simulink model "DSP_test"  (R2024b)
settings: Solver=VariableStepAuto  StartTime=0.0  StopTime=50  RelTol=1e-3
libraries: hdlsllib x1

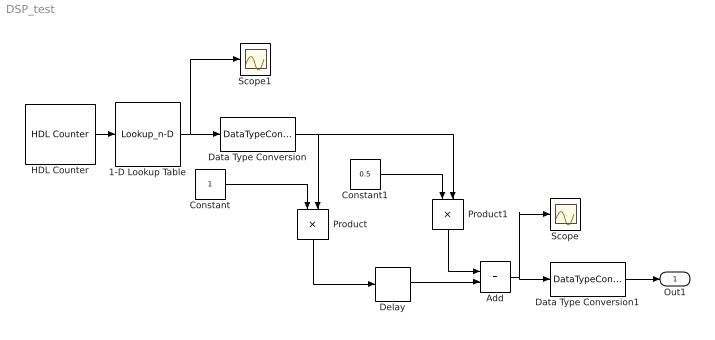
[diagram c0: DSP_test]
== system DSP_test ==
  1-D Lookup Table : Lookup_n-D  NumberOfTableDimensions=1  LookupTableObject=''  BreakpointsForDimension1=[0,1,2,3,4,5,6,7,8,9,10,11,12,13,14,15]  BreakpointsForDimension1FirstPoint=10  BreakpointsForDimension2FirstPoint=10  BreakpointsForDimension1Spacing=12  BreakpointsForDimension2Spacing=12  BreakpointsForDimension1Min=0  BreakpointsForDimension1Max=15  BreakpointsForDimension1DataTypeStr=uint8  IndexSearchMethod=Evenly spaced points  Table=[0,0.25,0.5,0.75,1,0.75,0.5,0.25,0,-0.25,-0.5,-0.75,-1,-0.75,-0.5,-0.25]  TableMin=-31  TableMax=31  TableDataTypeStr=fixdt(1,16,10)  InterpMethod=Flat  DiagnosticForOutOfRangeInput=Error  InternalRulePriority=Speed  OutMin=-31  OutMax=31  OutDataTypeStr=fixdt(1,16,10)  RndMeth=Simplest
  Add : Sum  OutMin=-31  OutMax=31  OutDataTypeStr=fixdt(1,16,0)  AccumDataTypeStr=fixdt(1,16,10)
  Constant : Constant  OutMin=-31  OutMax=31  OutDataTypeStr=fixdt(1,16,10)
  Constant1 : Constant  Value=0.5  OutMin=-31  OutMax=31  OutDataTypeStr=fixdt(1,16,10)
  Data Type Conversion : DataTypeConversion  OutMin=-31  OutMax=+31  OutDataTypeStr=fixdt(1,16,10)
  Data Type Conversion1 : DataTypeConversion  OutMin=-31  OutMax=31  OutDataTypeStr=fixdt(1,16,10)
  Delay : Delay  DelayLength=1  InitialCondition=0
  HDL Counter : hdlsllib/Sources/HDL Counter  CountType=Count limited  CountInit=0  CountStep=1  CountMax=15  CountFromType=Initial value  CountFrom=0  CountResetPort=off  CountLoadPort=off  CountEnbPort=off  CountDirPort=off  CountHitOutputPort=off  CountDataType=Unsigned  CountWordLen=4  CountFracLen=0  CountSampTime=1
  Product : Product  OutMin=-31  OutMax=31  OutDataTypeStr=fixdt(1,16,10)
  Product1 : Product  OutMin=-31  OutMax=31  OutDataTypeStr=fixdt(1,16,10)
  Scope : Scope
  Scope1 : Scope
  Out1 : Outport  OutMin=-31  OutMax=31  OutDataTypeStr=fixdt(1,16,10)  VectorParamsAs1DForOutWhenUnconnected=off
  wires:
  Constant/1 -> Product/1
  Product/1 -> Delay/1
  Add/1 -> Data Type Conversion1/1, Scope/1
  Delay/1 -> Add/2
  Product1/1 -> Add/1
  Constant1/1 -> Product1/1
  Data Type Conversion/1 -> Product/2, Product1/2
  1-D Lookup Table/1 -> Data Type Conversion/1, Scope1/1
  Data Type Conversion1/1 -> Out1/1
  HDL Counter/1 -> 1-D Lookup Table/1
